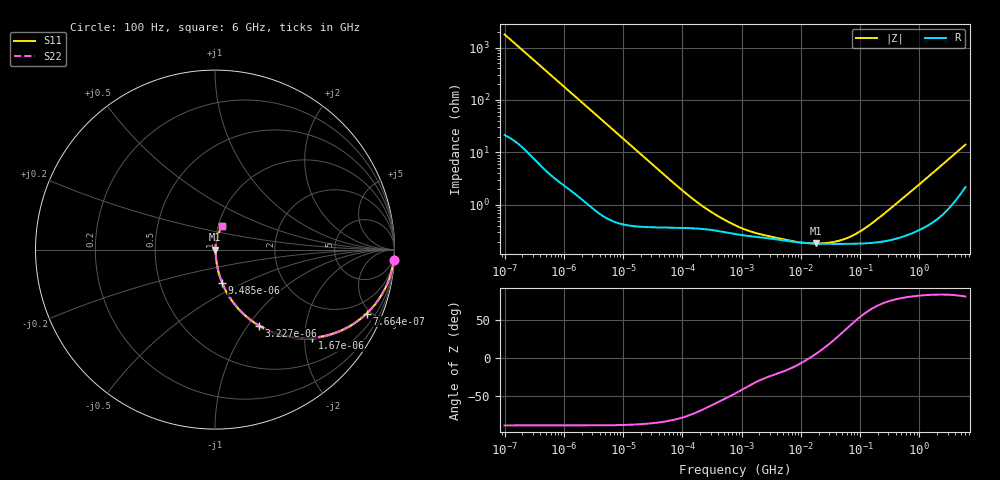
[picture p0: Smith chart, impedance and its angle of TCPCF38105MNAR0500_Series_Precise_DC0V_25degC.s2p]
! TCPCF38105MNAR0500 Polymer Tantalum Capacitor Sparameter Model
! Model Generated by Samsung Electro-Mechanics
! Samsung Sparameter Version 5.0
! Date : Oct-10-2024
! Products : Polymer Tantalum Capacitor
! Characteristics :
!  Nominal Capacitance = 1uF
!  Capacitance Tolerance = +/-20%
!  ESR = 500 mohm max at 100kHz
!  Rated Voltage = 38Vdc
!  Size = 0805(unit:inch), 2012(unit:mm)
!  Length = 2.00+/-0.20mm
!  Width = 1.25+/-0.20mm
!  Thickness = 0.80+/-0.10mm
!  Lineup = Conductive Polymer Type
!  Feature = PCF
!  Measurement Temperature : 25degC.
!  DC bias Value = 0V
!  Frequency : 100Hz ~ 6GHz
! External Node Assignments :
!  1  o---||---o  2
# MHz S RI R 50.0
! Freq.  Real(S11)  Im(S11)  Real(S12)  Im(S12)  Real(S21)  Im(S21)  Real(S22)  Im(S22)
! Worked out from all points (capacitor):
!   300 points, 100 Hz to 6 GHz, reference 50 ohm
!   read as one part in series: C = 895 nF near 106.2 Hz
!   lowest |Z| = 185 mohm at 17.98 MHz (marker M1)
!   series resonance near 14.2 MHz, so ESL is about 140 pH
!   S11 on the Smith chart (normalised r, x): 100 Hz: 1, -35; 766.4 Hz: 1.06, -4.71; 1.67 kHz: 1.03, -2.18; 3.227 kHz: 1.02, -1.13; 9.485 kHz: 1.01, -0.39; 6 GHz: 1.04, +0.28
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0.0001  0.9962 -0.0562  0.00385 0.0562  0.00385 0.0562  0.9962 -0.0562
0.0003517965  0.9608 -0.1876  0.0392 0.1876  0.0392 0.1876  0.9608 -0.1876
0.0007664292  0.8443 -0.3564  0.1557 0.3564  0.1557 0.3564  0.8443 -0.3564
0.001097881  0.7285 -0.4382  0.2715 0.4382  0.2715 0.4382  0.7285 -0.4382
0.001669754  0.5417 -0.4914  0.4583 0.4914  0.4583 0.4914  0.5417 -0.4914
0.001998454  0.4541 -0.4909  0.5459 0.4909  0.5459 0.4909  0.4541 -0.4909
0.003227047  0.2457 -0.4234  0.7543 0.4234  0.7543 0.4234  0.2457 -0.4234
0.005210943  0.1137 -0.3095  0.8863 0.3095  0.8863 0.3095  0.1137 -0.3095
0.009485389  0.0398 -0.1846  0.9602 0.1846  0.9602 0.1846  0.0398 -0.1846
0.03993819  0.0058 -0.0456  0.9942 0.0456  0.9942 0.0456  0.0058 -0.0456
0.2012627  0.0036 -0.0095  0.9964 0.0095  0.9964 0.0095  0.0036 -0.0095
0.7981464  0.00278 -0.00292  0.9972 0.00292  0.9972 0.00292  0.00278 -0.00292
2.346024  0.00237 -0.00123  0.9976 0.00123  0.9976 0.00123  0.00237 -0.00123
7.773385  0.00197 -0.000404  0.998 0.000404  0.998 0.000404  0.00197 -0.000404
15.95059  0.00184 8.24e-05  0.9982 -8.24e-05  0.9982 -8.24e-05  0.00184 8.24e-05
17.98061  0.00183 0.00017  0.9982 -0.00017  0.9982 -0.00017  0.00183 0.00017
36.89531  0.00181 0.000807  0.9982 -0.000807  0.9982 -0.000807  0.00181 0.000807
71.30563  0.00182 0.00177  0.9982 -0.00177  0.9982 -0.00177  0.00182 0.00177
129.7964  0.00187 0.00331  0.9981 -0.00331  0.9981 -0.00331  0.00187 0.00331
318.7652  0.00219 0.00808  0.9978 -0.00808  0.9978 -0.00808  0.00219 0.00808
1810.813  0.00674 0.0429  0.9933 -0.0429  0.9933 -0.0429  0.00674 0.0429
6000  0.0392 0.1308  0.9608 -0.1308  0.9608 -0.1308  0.0392 0.1308
